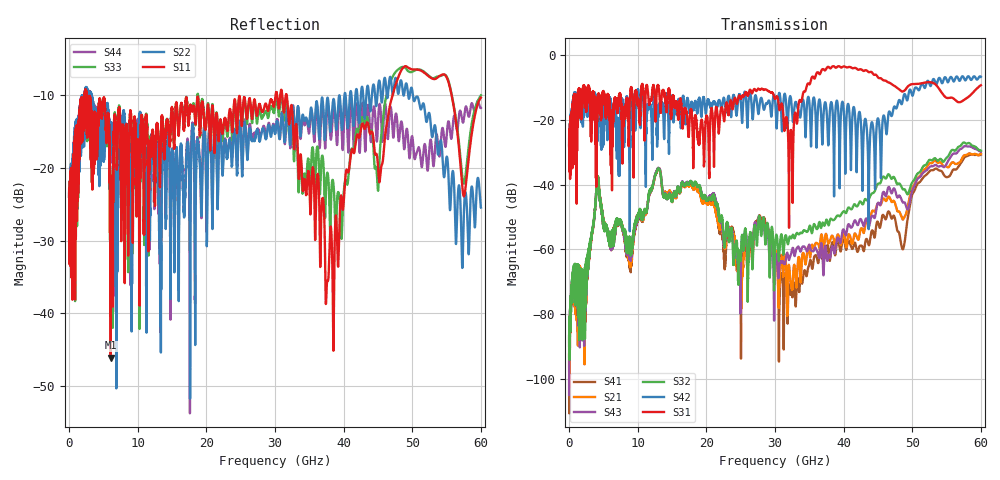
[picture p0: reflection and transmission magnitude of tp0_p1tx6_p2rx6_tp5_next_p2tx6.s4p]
! 100G CR Analysis
! File: tp0_p1tx6_p2rx6_tp5_next_p2tx6
! Description: 2m Cu Cable, OSFP, TP0-TP5
! Port Mapping
! Port1 -- P2TX6N
! Port2 -- P2RX6N
! Port3 -- P2TX6P
! Port4 -- P2RX6P
# GHz S MA R 50.00
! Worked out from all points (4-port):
!   6000 points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, 10 MHz to 60 GHz, reference 50 ohm
!   strongest paths, dB at 10 MHz, 15.01 GHz, 30.01 GHz, 45.01 GHz, 60 GHz:
!     S31: -28.2, -14.6, -13.5, -6.8, -9.3
!     S42: -27.9, -14.2, -13.6, -19.5, -6.7
!     S32: -87.6, -44.9, -59.7, -39.8, -29.5
!     S43: -105.1, -45.0, -64.2, -45.6, -29.9
!     S21: -86.8, -45.0, -61.4, -45.9, -30.4
!     S41: -92.6, -44.8, -63.4, -51.6, -30.7
!   lowest |S11| = -46.1 dB at 6.07 GHz (marker M1), VSWR 1.01, Z = 50.4 - j0.341 ohm
!   |S11| at or under -10 dB: 2.567 GHz to 30.08 GHz (27.51 GHz wide, 169 % of centre); 31.72 GHz to 47.12 GHz (15.4 GHz wide, 39.1 % of centre); 55.74 GHz to end of sweep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
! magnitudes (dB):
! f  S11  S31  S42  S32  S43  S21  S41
! 10 MHz  -24.0  -28.2  -27.9  -87.6  -105.1  -86.8  -92.6
! 4.17 GHz  -13.7  -12.8  -14.8  -37.4  -37.4  -37.3  -37.4
! 6.07 GHz  -46.1  -20.8  -14.0  -56.6  -57.2  -57.2  -57.3
! 13.02 GHz  -15.3  -9.6  -16.1  -35.1  -34.9  -35.2  -34.9
! 32.05 GHz  -14.0  -53.3  -14.6  -56.7  -63.3  -65.0  -70.9
! 37.61 GHz  -35.5  -3.7  -20.1  -51.2  -63.5  -56.7  -58.9
! 60 GHz  -10.3  -9.3  -6.7  -29.5  -29.9  -30.4  -30.7
